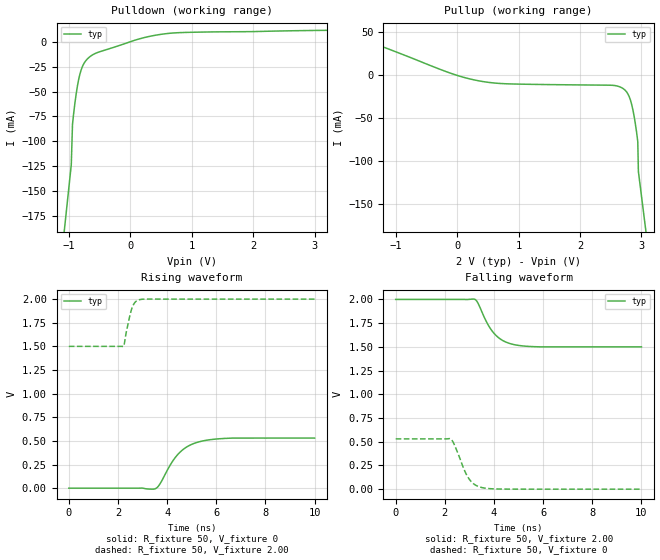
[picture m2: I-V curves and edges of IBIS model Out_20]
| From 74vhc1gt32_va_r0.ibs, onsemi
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|//////////////////////////////////////////////////////////////////////////////
|//////////////////////////////////////////////////////////////////////////////
[Model] Out_20
Model_type Output
Polarity Non-Inverting
Vmeas = 1.00
Vref = 2.00
Rref = 1k
Cref = 15pF
|  variable   typ   min   max
C_comp   3.9pF   3.9pF   3.9pF
|//////////////////////////////////////////////////////////////////////////////
[Temperature Range]   25   125   -55
|//////////////////////////////////////////////////////////////////////////////
[Voltage Range]   2.00V   NA   NA
|//////////////////////////////////////////////////////////////////////////////
[Pulldown Reference]   0V   NA   NA
|//////////////////////////////////////////////////////////////////////////////
[Pullup Reference]   2.00V   NA   NA
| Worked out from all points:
|   slope of the pulldown table from 0 to 0.3 V, typ, clamps not added: 57.6 ohm
|   slope of the pullup table from 0 to 0.3 V, typ, clamps not added: 53.7 ohm
|   falling waveform, R_fixture 50, V_fixture 2.00: 20-80 % time 714ps typ, NA min, NA max; typ from 2 V to 1.5 V
|   falling waveform, R_fixture 50, V_fixture 0: 20-80 % time 532ps typ, NA min, NA max; typ from 0.53 V to 0 V
|   rising waveform, R_fixture 50, V_fixture 0: 20-80 % time 888ps typ, NA min, NA max; typ from 0 V to 0.53 V
|   rising waveform, R_fixture 50, V_fixture 2.00: 20-80 % time 260ps typ, NA min, NA max; typ from 1.5 V to 2 V
|//////////////////////////////////////////////////////////////////////////////
[Pulldown]
|   Voltage   I(typ)   I(min)   I(max)
-2V       -736.8mA   NA         NA
-1.06V    -181.8mA   NA         NA
-960mV    -123.6mA   NA         NA
-940mV    -82.79mA   NA         NA
-900mV    -61.19mA   NA         NA
-860mV    -44.48mA   NA         NA
-820mV    -32.6mA    NA         NA
-760mV    -22.47mA   NA         NA
-600mV    -12.68mA   NA         NA
160mV     3.095mA    NA         NA
640mV     8.501mA    NA         NA
4V        11.92mA    NA         NA
|//////////////////////////////////////////////////////////////////////////////
[Pullup]
|   Voltage   I(typ)   I(min)   I(max)
-2V       54.4mA     NA         NA
280mV     -5.296mA   NA         NA
760mV     -9.631mA   NA         NA
2.5V      -11.45mA   NA         NA
2.68V     -14.42mA   NA         NA
2.8V      -24.63mA   NA         NA
2.84V     -33.54mA   NA         NA
2.88V     -47.22mA   NA         NA
2.94V     -76.88mA   NA         NA
2.95V     -111.7mA   NA         NA
3.06V     -174.2mA   NA         NA
4V        -708.6mA   NA         NA
|//////////////////////////////////////////////////////////////////////////////
|//////////////////////////////////////////////////////////////////////////////
[Ramp]
|  variable   typ   min   max
dV/dt_r   3.180E-01/9.000E-10  NA   NA
dV/dt_f   3.000E-01/7.000E-10  NA   NA
R_load = 50
|//////////////////////////////////////////////////////////////////////////////
[Falling Waveform]
R_fixture = 50
V_fixture = 2.00
C_fixture = 0p
|   time   V(typ)   V(min)   V(max)
0s        2V         NA         NA
3.2ns     2.003V     NA         NA
3.35ns    1.96V      NA         NA
3.7ns     1.761V     NA         NA
4ns       1.643V     NA         NA
4.2ns     1.594V     NA         NA
4.4ns     1.561V     NA         NA
4.9ns     1.519V     NA         NA
5.9ns     1.5V       NA         NA
10ns      1.5V       NA         NA
|//////////////////////////////////////////////////////////////////////////////
[Falling Waveform]
R_fixture = 50
V_fixture = 0
C_fixture = 0p
|   time   V(typ)   V(min)   V(max)
0s        530mV      NA         NA
2.225ns   530.3mV    NA         NA
2.3ns     511.4mV    NA         NA
2.375ns   475.4mV    NA         NA
2.775ns   212.4mV    NA         NA
2.95ns    121.9mV    NA         NA
3.2ns     50.94mV    NA         NA
3.525ns   15.92mV    NA         NA
4.5ns     678.4uV    NA         NA
10ns      0V         NA         NA
|//////////////////////////////////////////////////////////////////////////////
[Rising Waveform]
R_fixture = 50
V_fixture = 0
C_fixture = 0p
|   time   V(typ)   V(min)   V(max)
0s        0V         NA         NA
3.5ns     -7.809mV   NA         NA
3.6ns     8.2mV      NA         NA
3.7ns     41.49mV    NA         NA
4.15ns    255.4mV    NA         NA
4.5ns     374.6mV    NA         NA
4.9ns     450.9mV    NA         NA
5.45ns    499.7mV    NA         NA
6.65ns    529.7mV    NA         NA
10ns      530mV      NA         NA
|//////////////////////////////////////////////////////////////////////////////
[Rising Waveform]
R_fixture = 50
V_fixture = 2.00
C_fixture = 0p
|   time   V(typ)   V(min)   V(max)
0s        1.5V       NA         NA
2.225ns   1.499V     NA         NA
2.25ns    1.513V     NA         NA
2.325ns   1.632V     NA         NA
2.475ns   1.815V     NA         NA
2.575ns   1.908V     NA         NA
2.625ns   1.939V     NA         NA
2.7ns     1.968V     NA         NA
2.9ns     1.996V     NA         NA
10ns      2V         NA         NA
